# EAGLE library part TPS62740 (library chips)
360nA Step Down Converter for Low Power Applications
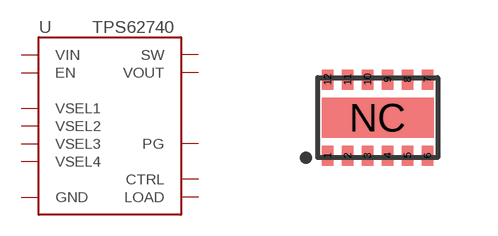
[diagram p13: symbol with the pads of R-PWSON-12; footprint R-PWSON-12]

Designator prefix U

## TPS62740 (DIGIKEY: 296-37134-1-ND; MOUSER: 595-TPS62740DSST; NEWARK: 27X9745)  [R-PWSON-12]
1  VIN
2  SW
3  GND
4  CTRL
5  VOUT
6  LOAD
7  PG
8  VSEL4
9  VSEL3
10  VSEL2
11  VSEL1
12  EN
NC  GND

## Footprint R-PWSON-12 (pad centres in mm)
smd 0.28 x 0.5: 1 -1.25,-0.95; 2 -0.75,-0.95; 3 -0.25,-0.95; 4 0.25,-0.95; 5 0.75,-0.95; 6 1.25,-0.95; 7 1.25,0.95; 8 0.75,0.95; 9 0.25,0.95; 10 -0.25,0.95; 11 -0.75,0.95; 12 -1.25,0.95
smd 2.8 x 1: NC 0,0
